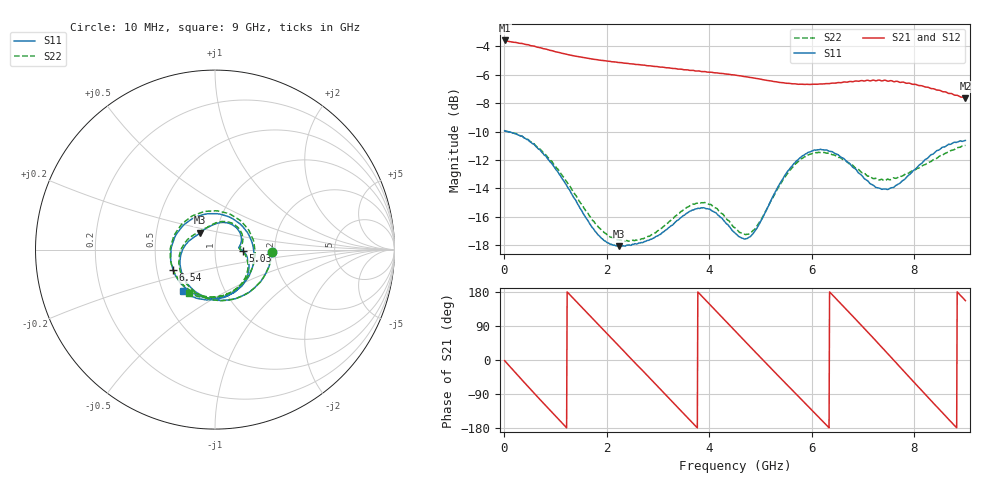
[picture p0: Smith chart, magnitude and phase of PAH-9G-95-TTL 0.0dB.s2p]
! MTS Systemtechnik GmbH
! S-Parameters
! Model: PAH-9G/95-TTL
! Attenuation Step: 0.0dB
#  HZ  S  DB  R  50.00
! Rohde & Schwarz Vector Network Analyzer
! Rohde-Schwarz,ZNB20-2Port,1334333062101652,3.45
! Created: UTC 1/26/2024, 7:16:40 AM
! freq[Hz]  db:S11  ang:S11  db:S21  ang:S21  db:S12  ang:S12  db:S22  ang:S22
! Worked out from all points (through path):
!   900 points, 10 MHz to 9 GHz, reference 50 ohm
!   highest |S21| = -3.59 dB at 10 MHz (marker M1); lowest = -7.7 dB at 9 GHz (marker M2)
!   group delay of S21, straight-line fit = 393 ps
!   lowest |S11| = -18.1 dB at 2.24 GHz (marker M3), VSWR 1.29, Z = 41.7 + j7.92 ohm
!   |S11| at or under -10 dB: 59.69 MHz to end of sweep
!   |S22| runs from -17.7 to -9.9 dB; largest |S21 - S12| = 0.018
!   S11 on the Smith chart (normalised r, x): 10 MHz: 1.93, -0.05; 5.03 GHz: 1.37, -0.02; 6.54 GHz: 0.61, -0.15; 9 GHz: 0.63, -0.32
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1e7  -9.95 -2.2  -3.59 -1.6  -3.60 -1.6  -9.94 -2.2
3.7e8  -10.39 -54.1  -3.83 -55.7  -3.83 -55.6  -10.38 -54.1
6.6e8  -11.20 -94.6  -4.07 -98.4  -4.08 -98.3  -11.15 -94.5
1.1e9  -13.12 -149.3  -4.47 -161.8  -4.47 -161.7  -12.91 -149.5
1.51e9  -15.54 171.2  -4.77 139.9  -4.78 140.0  -15.10 169.6
1.87e9  -17.40 148.3  -4.98 89.1  -4.99 89.2  -16.82 145.1
2.24e9  -18.07 131.4  -5.14 37.1  -5.15 37.0  -17.63 127.2
2.6e9  -17.90 115.4  -5.28 -14.0  -5.29 -13.5  -17.65 111.7
3.01e9  -17.32 97.2  -5.45 -71.8  -5.45 -71.7  -16.96 94.5
3.34e9  -16.39 80.3  -5.57 -118.6  -5.57 -118.0  -15.97 78.1
3.76e9  -15.44 52.9  -5.74 -177.7  -5.74 -177.3  -15.05 50.8
4.18e9  -15.90 23.6  -5.89 123.0  -5.90 123.3  -15.55 21.9
4.51e9  -17.17 8.0  -6.03 76.2  -6.03 76.6  -16.80 6.2
5.03e9  -16.17 -2.2  -6.34 2.8  -6.34 3.5  -16.10 -4.5
5.55e9  -12.73 -38.9  -6.60 -69.5  -6.63 -68.7  -12.83 -41.3
6.01e9  -11.37 -87.6  -6.67 -133.1  -6.70 -131.9  -11.54 -91.4
6.54e9  -11.71 -153.8  -6.56 152.9  -6.56 154.0  -11.83 -161.3
7.03e9  -13.33 133.3  -6.44 82.9  -6.42 84.1  -12.93 123.4
7.51e9  -14.03 50.3  -6.45 13.2  -6.43 14.1  -13.39 44.6
8.21e9  -11.99 -53.0  -6.87 -89.7  -6.87 -87.9  -12.34 -49.7
8.63e9  -11.00 -96.6  -7.24 -150.4  -7.30 -148.5  -11.49 -90.6
9e9  -10.63 -127.7  -7.65 156.6  -7.70 158.4  -10.97 -120.5
